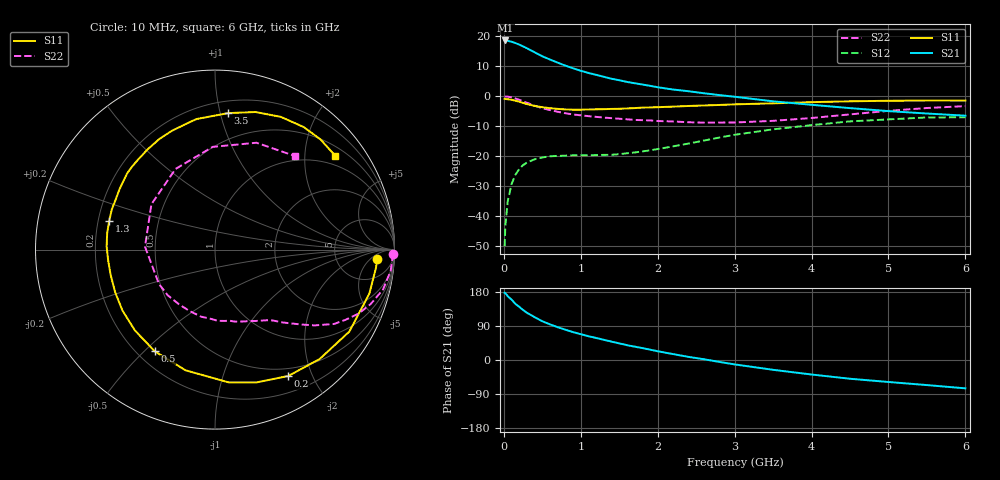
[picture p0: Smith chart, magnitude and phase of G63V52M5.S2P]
! SIEMENS Small Signal Semiconductors
! BFG193
! Si NPN RF Bipolar Junction Transistor in SOT223
! VCE = 3.5 V  IC = 2.5 mA
! Common Emitter S-Parameters:  August  1996
# GHz  S  MA  R  50
!  f  S11  S21  S12  S22
! GHz  MAG  ANG  MAG  ANG  MAG  ANG  MAG  ANG
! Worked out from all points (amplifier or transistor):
!   36 points, 10 MHz to 6 GHz, reference 50 ohm
!   highest |S21| = 18.6 dB at 20 MHz (marker M1)
!   |S21| within 3 dB of that: start of sweep to 329.9 MHz
!   unconditionally stable (mu >= 1): 1.316 GHz to 2.557 GHz
!   at 250 MHz: K = 0.21, MSG = 19.8 dB, |S12| = -22.9 dB
!   at 1.4 GHz: K = 1.06, MAG = 11.2 dB, |S12| = -19.5 dB
!   at 6 GHz: K = 0.94, MSG = 0.3 dB, |S12| = -7.0 dB
!   S11 on the Smith chart (normalised r, x): 10 MHz: 15, -9; 200 MHz: 0.40, -1.66; 500 MHz: 0.27, -0.54; 1.3 GHz: 0.25, +0.13; 3.5 GHz: 0.29, +1.06; 6 GHz: 0.72, +2.73
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0.01  0.9058 -3.3  8.406 177.5  0.0032 94.0  0.9943 -1.4
0.02  0.9025 -6.5  8.507 176.4  0.007 86.2  0.99 -2.7
0.05  0.8943 -15.9  8.392 168.4  0.0177 80.8  0.986 -6.9
0.1  0.8768 -31.4  8.099 159.4  0.0345 73.3  0.962 -13.4
0.15  0.8435 -46.3  7.704 148.3  0.0493 64.6  0.9187 -19.3
0.2  0.8138 -59.9  7.257 140.3  0.0615 58.7  0.875 -24.1
0.25  0.7753 -72.6  6.784 131.9  0.0715 52.4  0.8244 -28.4
0.3  0.7434 -84.2  6.306 124.7  0.0789 47.5  0.7818 -32.0
0.4  0.6922 -103.7  5.408 113.1  0.0894 39.4  0.6969 -37.3
0.5  0.6586 -120.6  4.632 102.3  0.0958 33.6  0.6346 -41.1
0.6  0.634 -134.7  4.094 94.1  0.1002 29.7  0.5898 -44.2
0.7  0.6173 -146.7  3.639 86.5  0.102 26.9  0.553 -47.2
0.9  0.5983 -166.5  2.923 73.6  0.1042 23.8  0.4992 -51.9
1.1  0.604 178.3  2.448 62.8  0.1046 23.4  0.4674 -58.0
1.3  0.6109 164.8  2.115 53.3  0.1059 24.4  0.4423 -63.9
1.6  0.6283 148.3  1.736 39.2  0.1126 27.9  0.4148 -75.0
2.2  0.6732 123.8  1.296 15.6  0.1469 32.9  0.3815 -101.8
2.8  0.7175 103.5  1.049 -5.0  0.2058 29.0  0.366 -136.0
3.5  0.7639 84.5  0.825 -25.9  0.2819 14.8  0.3904 177.6
4.5  0.8255 63.6  0.636 -49.5  0.3824 -8.3  0.5003 116.1
5.5  0.85 46.2  0.517 -66.2  0.4446 -36.6  0.6386 68.8
6  0.8494 38.1  0.476 -74.8  0.4478 -51.8  0.6866 49.3
